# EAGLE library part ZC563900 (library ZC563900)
NodeMcu Lua ESP8266 WIFI Internet of Things Network Development Module Board Check availability
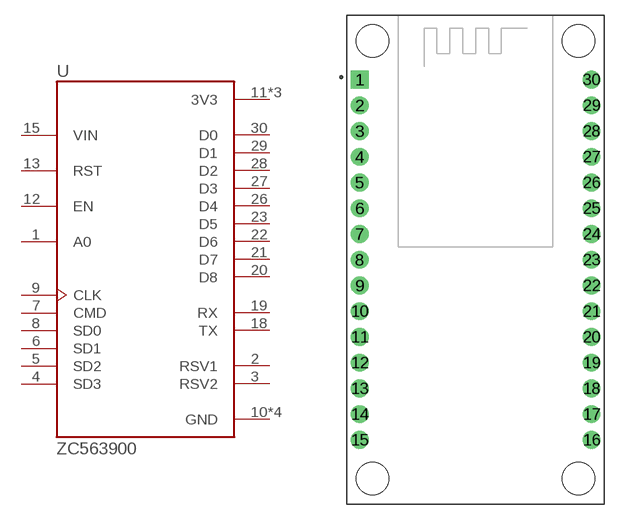
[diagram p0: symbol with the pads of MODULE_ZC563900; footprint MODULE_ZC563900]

Designator prefix U

## ZC563900 (Availability: Not in stock; Description: NodeMcu Lua ESP8266 WIFI Internet of Things Network Development Module Board; MF: YKS; MP: ZC563900; Package: None; Price: None)  [MODULE_ZC563900]
1  A0  in
2  RSV1  pas
3  RSV2  pas
4  SD3
5  SD2
6  SD1
7  CMD  in
8  SD0
9  CLK  in
10  GND  pwr
11  3V3  pwr
12  EN  in
13  RST  in
14  GND  pwr
15  VIN  in
16  3V3  pwr
17  GND  pwr
18  TX
19  RX
20  D8
21  D7
22  D6
23  D5
24  GND  pwr
25  3V3  pwr
26  D4
27  D3
28  D2
29  D1
30  D0

## Footprint MODULE_ZC563900 (pad centres in mm)
drill 0.889 pad 1.753 square: 1 -11.43,17.78
drill 0.889 pad 1.753: 2 -11.43,15.24; 3 -11.43,12.7; 4 -11.43,10.16; 5 -11.43,7.62; 6 -11.43,5.08; 7 -11.43,2.54; 8 -11.43,0; 9 -11.43,-2.54; 10 -11.43,-5.08; 11 -11.43,-7.62; 12 -11.43,-10.16; 13 -11.43,-12.7; 14 -11.43,-15.24; 15 -11.43,-17.78; 16 11.43,-17.78; 17 11.43,-15.24; 18 11.43,-12.7; 19 11.43,-10.16; 20 11.43,-7.62; 21 11.43,-5.08; 22 11.43,-2.54; 23 11.43,0; 24 11.43,2.54; 25 11.43,5.08; 26 11.43,7.62; 27 11.43,10.16; 28 11.43,12.7; 29 11.43,15.24; 30 11.43,17.78
hole 3.2 at -10.16,21.59
hole 3.2 at 10.16,21.59
hole 3.2 at 10.16,-21.59
hole 3.2 at -10.16,-21.59

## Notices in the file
This work is licensed under a Creative Commons Attribution-ShareAlike 4.0 International License (CC BY-SA) with Design Exception 1.0
